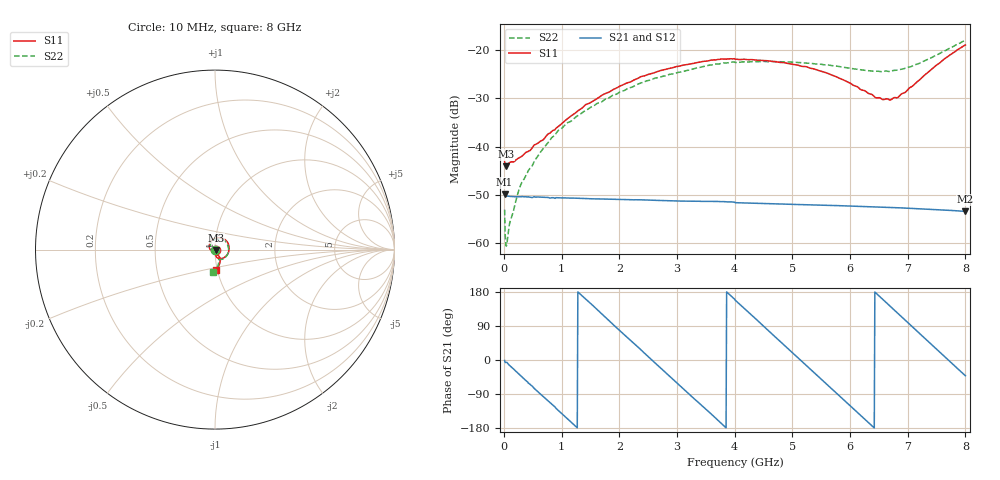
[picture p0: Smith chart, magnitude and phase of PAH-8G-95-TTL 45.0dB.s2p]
! MTS Systemtechnik GmbH
! S-Parameters
! Model: PAH-8G/95-TTL
! Attenuation Step: 45.0dB
! Rohde & Schwarz ZVB8 2Ports - Version 4.11 - 1145.1010k08 SN: 100119
! S2P File Measurements:
! S11 S21 S12 S22
# HZ  S  DB  R  50.00
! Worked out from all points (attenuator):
!   800 points, 10 MHz to 8 GHz, reference 50 ohm
!   highest |S21| = -49.91 dB at 10 MHz (marker M1); lowest = -53.4 dB at 8 GHz (marker M2)
!   lowest |S11| = -44.1 dB at 30 MHz (marker M3), VSWR 1.01, Z = 50.6 - j0.135 ohm
!   |S11| at or under -10 dB: start of sweep to end of sweep
!   |S22| runs from -60.6 to -18.0 dB; largest |S21 - S12| = 4.5e-05
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1e7  -43.08 -18.4  -49.91 -1.3  -49.81 -1.1  -53.08 -80.4
3e7  -44.07 -12.3  -50.31 -6.4  -50.33 -6.4  -60.32 -78.9
6e7  -43.78 -12.2  -50.26 -8.3  -50.28 -8.1  -59.22 -64.0
7e7  -43.64 -14.1  -50.29 -10.2  -50.30 -10.1  -58.21 -62.2
1.3e8  -43.16 -23.1  -50.35 -19.1  -50.36 -19.1  -54.64 -69.3
2.9e8  -42.18 -50.0  -50.42 -41.7  -50.43 -41.7  -47.93 -93.9
5.6e8  -39.49 -89.7  -50.45 -80.2  -50.49 -79.9  -42.40 -122.9
9.4e8  -35.85 -135.7  -50.62 -132.9  -50.61 -132.9  -36.69 -153.4
1.35e9  -32.08 -174.3  -50.75 169.9  -50.76 169.9  -33.04 178.7
2.01e9  -27.48 138.3  -50.95 77.2  -50.98 77.5  -28.67 136.8
2.68e9  -24.38 97.3  -51.17 -16.4  -51.16 -16.1  -25.71 100.3
3.44e9  -22.40 54.5  -51.35 -121.5  -51.37 -121.9  -23.48 60.0
4.01e9  -21.92 21.9  -51.63 157.6  -51.63 157.5  -22.60 30.1
4.69e9  -22.37 -15.3  -51.87 62.7  -51.89 62.7  -22.42 -3.6
5.34e9  -23.85 -49.4  -52.09 -27.9  -52.11 -27.9  -22.80 -33.7
5.89e9  -26.23 -73.2  -52.28 -104.9  -52.30 -105.0  -23.59 -54.7
6.45e9  -29.89 -80.4  -52.51 176.5  -52.52 176.4  -24.40 -67.8
6.67e9  -30.26 -71.9  -52.60 145.5  -52.61 145.5  -24.45 -69.5
6.82e9  -29.88 -65.8  -52.67 124.4  -52.69 124.3  -24.15 -70.8
6.95e9  -28.83 -61.3  -52.75 106.0  -52.76 106.0  -23.80 -71.8
7.62e9  -21.98 -70.1  -53.14 11.7  -53.16 11.7  -20.32 -81.6
8e9  -18.96 -87.5  -53.44 -41.6  -53.47 -41.4  -18.03 -94.6
